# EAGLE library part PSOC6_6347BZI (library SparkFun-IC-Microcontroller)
PSoC6 with Dual core M0+, M4, BLE 1MB Flash, 288k SRAM, BGA-116 pkg
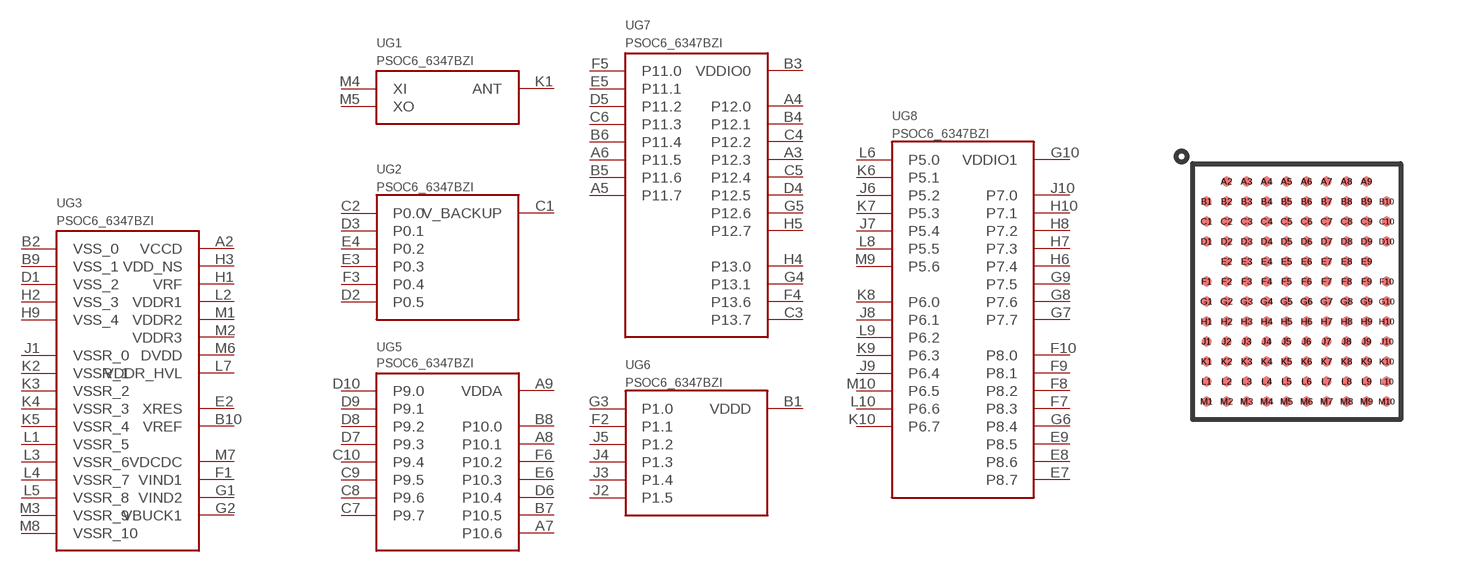
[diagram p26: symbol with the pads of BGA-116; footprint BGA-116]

Designator prefix U; gates G1=CY8C6347BZI_ASST G2=CY8C6347BZI_P0_P1 G3=CY8C6347BZI_SUPPLY G5=CY8C6347BZI_VDDA G6=CY8C6347BZI_VDDD G7=CY8C6347BZI_VDDIO0 G8=CY8C6347BZI_VDDIO1

## PSOC6_6347BZI (VALUE: CY8C6347BZI)  [BGA-116]
A2  G3:VCCD
A3  G7:P12.3
A4  G7:P12.0
A5  G7:P11.7
A6  G7:P11.5
A7  G5:P10.6
A8  G5:P10.1
A9  G5:VDDA
B1  G6:VDDD
B2  G3:VSS_0
B3  G7:VDDIO0
B4  G7:P12.1
B5  G7:P11.6
B6  G7:P11.4
B7  G5:P10.5
B8  G5:P10.0
B9  G3:VSS_1
B10  G3:VREF
C1  G2:V_BACKUP
C2  G2:P0.0
C3  G7:P13.7
C4  G7:P12.2
C5  G7:P12.4
C6  G7:P11.3
C7  G5:P9.7
C8  G5:P9.6
C9  G5:P9.5
C10  G5:P9.4
D1  G3:VSS_2
D2  G2:P0.5
D3  G2:P0.1
D4  G7:P12.5
D5  G7:P11.2
D6  G5:P10.4
D7  G5:P9.3
D8  G5:P9.2
D9  G5:P9.1
D10  G5:P9.0
E2  G3:XRES
E3  G2:P0.3
E4  G2:P0.2
E5  G7:P11.1
E6  G5:P10.3
E7  G8:P8.7
E8  G8:P8.6
E9  G8:P8.5
F1  G3:VIND1
F2  G6:P1.1
F3  G2:P0.4
F4  G7:P13.6
F5  G7:P11.0
F6  G5:P10.2
F7  G8:P8.3
F8  G8:P8.2
F9  G8:P8.1
F10  G8:P8.0
G1  G3:VIND2
G2  G3:VBUCK1
G3  G6:P1.0
G4  G7:P13.1
G5  G7:P12.6
G6  G8:P8.4
G7  G8:P7.7
G8  G8:P7.6
G9  G8:P7.5
G10  G8:VDDIO1
H1  G3:VRF
H2  G3:VSS_3
H3  G3:VDD_NS
H4  G7:P13.0
H5  G7:P12.7
H6  G8:P7.4
H7  G8:P7.3
H8  G8:P7.2
H9  G3:VSS_4
H10  G8:P7.1
J1  G3:VSSR_0
J2  G6:P1.5
J3  G6:P1.4
J4  G6:P1.3
J5  G6:P1.2
J6  G8:P5.2
J7  G8:P5.4
J8  G8:P6.1
J9  G8:P6.4
J10  G8:P7.0
K1  G1:ANT
K2  G3:VSSR_1
K3  G3:VSSR_2
K4  G3:VSSR_3
K5  G3:VSSR_4
K6  G8:P5.1
K7  G8:P5.3
K8  G8:P6.0
K9  G8:P6.3
K10  G8:P6.7
L1  G3:VSSR_5
L2  G3:VDDR1
L3  G3:VSSR_6
L4  G3:VSSR_7
L5  G3:VSSR_8
L6  G8:P5.0
L7  G3:VDDR_HVL
L8  G8:P5.5
L9  G8:P6.2
L10  G8:P6.6
M1  G3:VDDR2
M2  G3:VDDR3
M3  G3:VSSR_9
M4  G1:XI
M5  G1:XO
M6  G3:DVDD
M7  G3:VDCDC
M8  G3:VSSR_10
M9  G8:P5.6
M10  G8:P6.5

## Footprint BGA-116 (pad centres in mm)
smd 0.25 x 0.25: A2 -1.75,2.75; A3 -1.25,2.75; A4 -0.75,2.75; A5 -0.25,2.75; A6 0.25,2.75; A7 0.75,2.75; A8 1.25,2.75; A9 1.75,2.75; B1 -2.25,2.25; B2 -1.75,2.25; B3 -1.25,2.25; B4 -0.75,2.25; B5 -0.25,2.25; B6 0.25,2.25; B7 0.75,2.25; B8 1.25,2.25; B9 1.75,2.25; B10 2.25,2.25; C1 -2.25,1.75; C2 -1.75,1.75; C3 -1.25,1.75; C4 -0.75,1.75; C5 -0.25,1.75; C6 0.25,1.75; C7 0.75,1.75; C8 1.25,1.75; C9 1.75,1.75; C10 2.25,1.75; D1 -2.25,1.25; D2 -1.75,1.25; D3 -1.25,1.25; D4 -0.75,1.25; D5 -0.25,1.25; D6 0.25,1.25; D7 0.75,1.25; D8 1.25,1.25; D9 1.75,1.25; D10 2.25,1.25; E2 -1.75,0.75; E3 -1.25,0.75; E4 -0.75,0.75; E5 -0.25,0.75; E6 0.25,0.75; E7 0.75,0.75; E8 1.25,0.75; E9 1.75,0.75; F1 -2.25,0.25; F2 -1.75,0.25; F3 -1.25,0.25; F4 -0.75,0.25; F5 -0.25,0.25; F6 0.25,0.25; F7 0.75,0.25; F8 1.25,0.25; F9 1.75,0.25; F10 2.25,0.25; G1 -2.25,-0.25; G2 -1.75,-0.25; G3 -1.25,-0.25; G4 -0.75,-0.25; G5 -0.25,-0.25; G6 0.25,-0.25; G7 0.75,-0.25; G8 1.25,-0.25; G9 1.75,-0.25; G10 2.25,-0.25; H1 -2.25,-0.75; H2 -1.75,-0.75; H3 -1.25,-0.75; H4 -0.75,-0.75; H5 -0.25,-0.75; H6 0.25,-0.75; H7 0.75,-0.75; H8 1.25,-0.75; H9 1.75,-0.75; H10 2.25,-0.75; J1 -2.25,-1.25; J2 -1.75,-1.25; J3 -1.25,-1.25; J4 -0.75,-1.25; J5 -0.25,-1.25; J6 0.25,-1.25; J7 0.75,-1.25; J8 1.25,-1.25; J9 1.75,-1.25; J10 2.25,-1.25; K1 -2.25,-1.75; K2 -1.75,-1.75; K3 -1.25,-1.75; K4 -0.75,-1.75; K5 -0.25,-1.75; K6 0.25,-1.75; K7 0.75,-1.75; K8 1.25,-1.75; K9 1.75,-1.75; K10 2.25,-1.75; L1 -2.25,-2.25; L2 -1.75,-2.25; L3 -1.25,-2.25; L4 -0.75,-2.25; L5 -0.25,-2.25; L6 0.25,-2.25; L7 0.75,-2.25; L8 1.25,-2.25; L9 1.75,-2.25; L10 2.25,-2.25; M1 -2.25,-2.75; M2 -1.75,-2.75; M3 -1.25,-2.75; M4 -0.75,-2.75; M5 -0.25,-2.75; M6 0.25,-2.75; M7 0.75,-2.75; M8 1.25,-2.75; M9 1.75,-2.75; M10 2.25,-2.75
